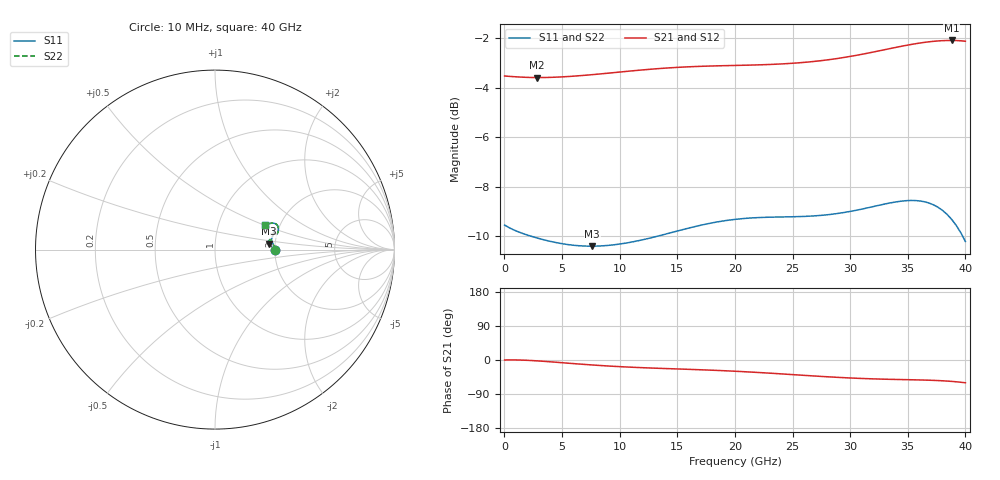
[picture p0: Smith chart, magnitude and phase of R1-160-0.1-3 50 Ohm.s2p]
!version-1
!date-09.2020
# MHz S RI R 50
!Freq ReS11 ImS11 ReS21 ImS21 ReS12 ImS12 ReS22 ImS22
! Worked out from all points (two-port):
!   101 points, 10 MHz to 40 GHz, reference 50 ohm
!   highest |S21| = -2.09 dB at 38.81 GHz (marker M1); lowest = -3.6 dB at 2.81 GHz (marker M2)
!   |S21| within 3 dB of the highest: start of sweep to end of sweep
!   lowest |S11| = -10.4 dB at 7.61 GHz (marker M3), VSWR 1.87, Z = 92.6 + j6.75 ohm
!   |S11| at or under -10 dB: 2.334 GHz to 13.24 GHz (10.91 GHz wide, 140 % of centre); 39.76 GHz to end of sweep
!   |S22| runs from -10.4 to -8.6 dB; largest |S21 - S12| = 0
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10  0.3332 0.000458  0.6666 9.83e-05  0.6666 9.83e-05  0.3332 0.000458
410  0.3287 0.0168  0.6656 0.00253  0.6656 0.00253  0.3287 0.0168
1210  0.3204 0.0392  0.6637 -0.000127  0.6637 -0.000127  0.3204 0.0392
2010  0.3138 0.0512  0.6623 -0.0105  0.6623 -0.0105  0.3138 0.0512
2810  0.3088 0.0558  0.6614 -0.0261  0.6614 -0.0261  0.3088 0.0558
4010  0.304 0.0541  0.6601 -0.0557  0.6601 -0.0557  0.304 0.0541
6810  0.3 0.037  0.6553 -0.1319  0.6553 -0.1319  0.3 0.037
7610  0.3002 0.0331  0.6533 -0.1522  0.6533 -0.1522  0.3002 0.0331
10410  0.3044 0.032  0.6466 -0.212  0.6466 -0.212  0.3044 0.032
13610  0.3135 0.0522  0.6396 -0.2605  0.6396 -0.2605  0.3135 0.0522
17210  0.3231 0.083  0.627 -0.3057  0.627 -0.3057  0.3231 0.083
20010  0.3279 0.0975  0.6084 -0.3466  0.6084 -0.3466  0.3279 0.0975
22810  0.3312 0.0986  0.5804 -0.3968  0.5804 -0.3968  0.3312 0.0986
26810  0.3365 0.0875  0.5296 -0.4777  0.5296 -0.4777  0.3365 0.0875
30410  0.3456 0.0878  0.4908 -0.5445  0.4908 -0.5445  0.3456 0.0878
33610  0.3531 0.1099  0.4765 -0.5903  0.4765 -0.5903  0.3531 0.1099
35210  0.3514 0.1268  0.474 -0.6086  0.474 -0.6086  0.3514 0.1268
36810  0.3411 0.1417  0.467 -0.6266  0.467 -0.6266  0.3411 0.1417
38010  0.325 0.1473  0.4523 -0.6426  0.4523 -0.6426  0.325 0.1473
38810  0.3093 0.1463  0.4344 -0.6557  0.4344 -0.6557  0.3093 0.1463
39610  0.2888 0.1407  0.4075 -0.6712  0.4075 -0.6712  0.2888 0.1407
40000  0.2771 0.1361  0.3904 -0.6797  0.3904 -0.6797  0.2771 0.1361
